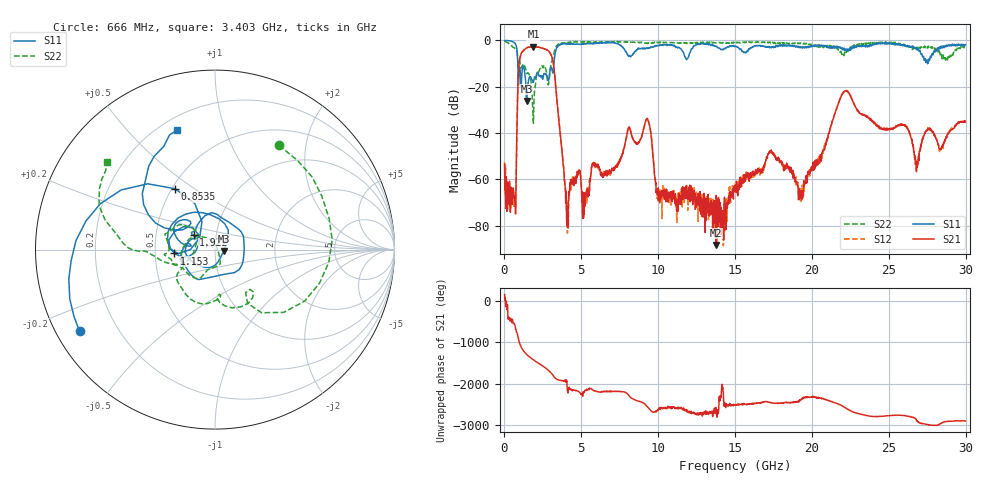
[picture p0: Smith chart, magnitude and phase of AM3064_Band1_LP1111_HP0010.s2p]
# Hz S DB R 50.0
!freq dBS11 angS11 dBS21 angS21 dBS12 angS12 dBS22 angS22
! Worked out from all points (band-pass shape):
!   1600 points, 10 MHz to 29.98 GHz, reference 50 ohm
!   highest |S21| = -2.67 dB at 1.884 GHz (marker M1); lowest = -88.3 dB at 13.75 GHz (marker M2)
!   |S21| within 3 dB of the highest: 1.09 GHz to 2.99 GHz (1.9 GHz wide, 93.1 % of centre)
!   lowest |S11| = -26.1 dB at 1.435 GHz (marker M3), VSWR 1.10, Z = 55.1 - j0.872 ohm
!   |S11| at or under -10 dB: 866.1 MHz to 3.218 GHz (2.352 GHz wide, 115 % of centre); 27.52402 GHz to 27.53223 GHz (8.208 MHz wide, 0.0298 % of centre)
!   |S22| runs from -35.8 to -0.2 dB; largest |S21 - S12| = 0.012
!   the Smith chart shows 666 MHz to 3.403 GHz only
!   S11 on the Smith chart (normalised r, x): 666 MHz: 0.07, -0.28; 853.5 MHz: 0.52, +0.42; 1.153 GHz: 0.63, -0.03; 1.922 GHz: 0.78, +0.13; 3.403 GHz: 0.27, +0.70
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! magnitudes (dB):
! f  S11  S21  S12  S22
! 10 MHz  -0.1  -53.5  -52.6  -0.2
! 666 MHz  -1.1  -69.2  -65.1  -3.3
! 853.5 MHz  -7.9  -24.7  -24.7  -7.2
! 1.153 GHz  -12.9  -5.0  -4.9  -11.1
! 1.435 GHz  -26.1  -3.3  -3.2  -14.2
! 1.884 GHz  -17.9  -2.7  -2.7  -35.8
! 1.922 GHz  -16.8  -2.7  -2.7  -25.7
! 3.009 GHz  -11.9  -5.9  -5.9  -10.9
! 3.403 GHz  -3.1  -25.0  -24.9  -2.2
! 4.059 GHz  -1.3  -79.6  -70.6  -1.0
! 5.015 GHz  -1.4  -64.8  -64.0  -0.6
! 9.288 GHz  -3.5  -33.9  -33.8  -1.3
! 10 GHz  -2.2  -63.6  -66.1  -0.9
! 13.75 GHz  -2.5  -88.3  -80.4  -1.0
! 15 GHz  -2.5  -62.5  -61.5  -1.2
! 17.27 GHz  -3.0  -47.7  -48.1  -1.0
! 19.28 GHz  -3.2  -64.9  -68.6  -1.2
! 19.99 GHz  -2.8  -56.1  -56.6  -1.8
! 22.15 GHz  -4.5  -21.8  -21.7  -5.2
! 25 GHz  -1.1  -38.5  -37.5  -1.0
! 26.81 GHz  -3.5  -53.7  -52.8  -3.7
! 29.98 GHz  -1.9  -35.0  -35.3  -2.8
